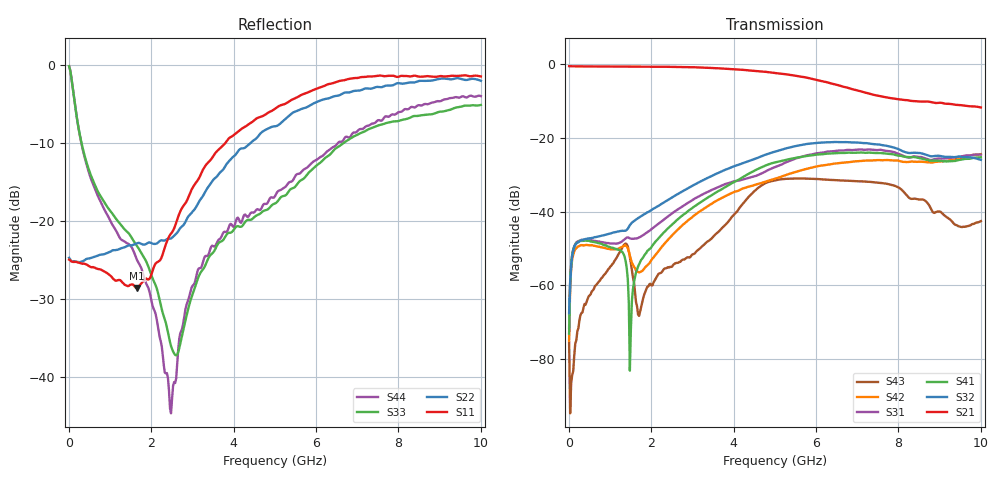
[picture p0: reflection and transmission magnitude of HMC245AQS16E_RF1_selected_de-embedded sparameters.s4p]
! Device:	HMC245AQS16E
! Description:	GaAs MMIC SP3T Non-Reflective Switch
! Package:	LP3E - 16 pin 3x3mm QFN plastic package
! Frequency:	DC -  3.5 GHz
! Ports:
! RFC = Port 1
! RF1 = Port 2
! RF2 = Port 3
! RF3 = Port 4
! State: RF1 Selected
! Supply Voltage:
! Vdd = 5 V
! Control Voltages:
! VA  = 0 V
! VB  = 0 V
! Data:	Data was collected using a calibrated network analyzer with AFR software.
!	Fixtures were calculated using AFR and fixturing was applied to collect
!	this Deembedded  S Parameter data of HMC245AQS16E
! Note:	Analog Devices supplies this data as a sample of measured data at the package pin
!	for this product.  Your particular data for this product may vary.
!	Data was taken at 25 degrees C.
!	Analog Devices reserves the right to change this data at anytime.
# GHz S  dB  R 50
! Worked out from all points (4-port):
!   401 points, 10 MHz to 10 GHz, reference 50 ohm
!   strongest paths, dB at 10 MHz, 2.507 GHz, 5.005 GHz, 7.503 GHz, 10 GHz:
!     S21: -0.6, -0.8, -2.4, -8.6, -11.8
!     S32: -67.6, -36.2, -23.8, -21.8, -26.0
!     S41: -73.1, -43.5, -26.7, -24.1, -25.3
!     S31: -71.6, -40.5, -28.0, -23.3, -24.6
!     S42: -75.0, -46.5, -31.1, -26.0, -24.4
!     S43: -75.6, -55.0, -31.6, -32.2, -42.6
!   lowest |S11| = -28.6 dB at 1.658 GHz (marker M1), VSWR 1.08, Z = 50.4 - j3.71 ohm
!   |S11| at or under -10 dB: start of sweep to 3.804 GHz
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0.01  -24.97 -1.4  -0.57 -0.4  -73.16 84.5  -78.84 106.1
      -0.57 -0.4  -24.74 -0.7  -72.94 69.7  -69.42 122.6
      -71.60 118.7  -67.58 70.4  -0.18 -5.7  -90.91 146.1
      -73.11 110.0  -75.05 134.8  -75.60 -120.1  -0.18 -5.8
0.2098  -25.31 -9.7  -0.62 -6.4  -48.27 18.8  -48.34 31.5
        -0.63 -6.4  -25.27 -6.3  -48.48 41.1  -49.65 24.4
        -48.17 18.7  -48.43 41.5  -7.20 -60.2  -72.91 113.0
        -48.48 30.9  -49.65 24.0  -72.45 132.6  -7.24 -60.3
1.35865  -28.19 -59.4  -0.69 -40.5  -47.48 -93.8  -52.40 -19.7
         -0.69 -40.5  -23.38 -32.2  -45.21 73.7  -49.22 -82.0
         -47.50 -94.0  -45.21 73.8  -21.11 -67.5  -48.79 40.2
         -52.33 -19.8  -49.23 -82.1  -48.81 40.1  -22.66 -64.8
1.65835  -28.61 -82.3  -0.69 -49.5  -47.27 -136.6  -55.75 102.2
         -0.70 -49.5  -22.87 -43.2  -41.99 86.5  -56.37 -148.2
         -47.26 -136.8  -41.99 86.5  -23.22 -68.2  -66.16 3.1
         -55.70 102.3  -56.24 -149.4  -65.75 1.6  -25.03 -70.7
2.482525  -21.64 -154.2  -0.75 -75.3  -40.71 160.8  -43.77 108.3
          -0.75 -75.3  -22.26 -95.4  -36.38 94.2  -46.76 143.5
          -40.71 160.8  -36.37 94.2  -36.04 -112.8  -55.00 94.0
          -43.77 108.5  -46.76 143.7  -55.03 93.9  -44.67 -163.2
4.880125  -6.02 105.9  -2.23 -155.8  -28.51 65.7  -27.06 43.1
          -2.24 -155.8  -8.06 123.1  -24.16 53.5  -31.52 46.9
          -28.52 65.7  -24.16 53.5  -18.27 113.5  -31.86 60.9
          -27.08 43.1  -31.51 46.8  -31.86 60.8  -17.11 89.4
10  -1.49 -27.6  -11.77 66.9  -24.56 -104.1  -25.27 -112.4
    -11.77 67.0  -2.05 -17.6  -25.98 -86.9  -24.43 -116.1
    -24.56 -104.1  -25.99 -87.0  -5.14 -0.6  -42.68 160.3
    -25.28 -112.4  -24.43 -116.0  -42.60 161.1  -4.02 -13.5
